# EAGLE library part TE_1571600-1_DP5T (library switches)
Through hole DP5T switch.
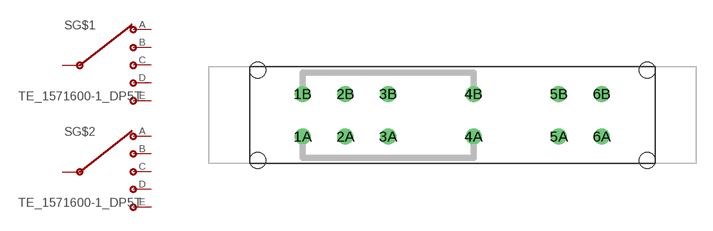
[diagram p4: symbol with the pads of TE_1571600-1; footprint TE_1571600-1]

Designator prefix S; gates G$1=SP5T G$2=SP5T

## TE_1571600-1_DP5T (DIGIKEY: A112404-ND)  [TE_1571600-1]
1A  G$1:A
1B  G$2:A
2A  G$1:B
2B  G$2:B
3A  G$1:C
3B  G$2:C
4A  G$1:INPUT
4B  G$2:INPUT
5A  G$1:D
5B  G$2:D
6A  G$1:E
6B  G$2:E

## Footprint TE_1571600-1 (pad centres in mm)
DP5T
drill 0.8 pad 1.5: 1A -14.03,-2; 1B -14.03,2; 2A -10.03,-2; 2B -10.03,2; 3A -6.03,-2; 3B -6.03,2; 4A 1.97,-2; 4B 1.97,2; 5A 9.97,-2; 5B 9.97,2; 6A 13.97,-2; 6B 13.97,2
hole 1.5 at 18.25,4.25
hole 1.5 at 18.25,-4.25
hole 1.5 at -18.25,4.25
hole 1.5 at -18.25,-4.25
